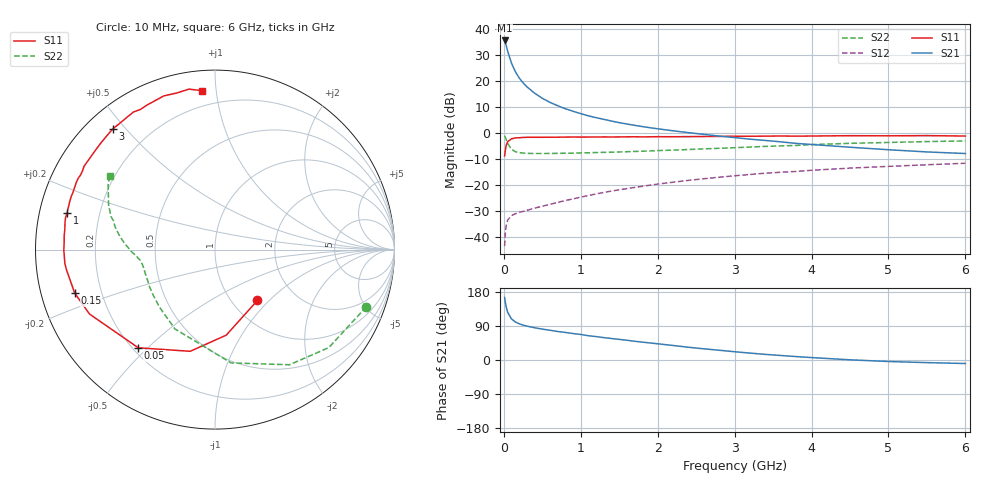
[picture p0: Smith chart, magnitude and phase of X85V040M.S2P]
! SIEMENS Small Signal Semiconductors
! BFP136W
! Si NPN RF Bipolar Junction Transistor in SOT343
! VCE = 5 V  IC = 40 mA
! Common Emitter S-Parameters:  September  1994
# GHz  S  MA  R  50
!  f  S11  S21  S12  S22
! GHz  MAG  ANG  MAG  ANG  MAG  ANG  MAG  ANG
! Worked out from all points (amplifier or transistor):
!   40 points, 10 MHz to 6 GHz, reference 50 ohm
!   highest |S21| = 35.7 dB at 10 MHz (marker M1)
!   |S21| within 3 dB of that: start of sweep to 40.07 MHz
!   unconditionally stable (mu >= 1): 746.3 MHz to 2.851 GHz
!   at 200 MHz: K = 0.48, MSG = 25.8 dB, |S12| = -30.4 dB
!   at 1.5 GHz: K = 1.11, MAG = 10.8 dB, |S12| = -21.7 dB
!   at 6 GHz: K = 0.96, MSG = 1.9 dB, |S12| = -11.5 dB
!   S11 on the Smith chart (normalised r, x): 10 MHz: 1.30, -0.85; 50 MHz: 0.22, -0.47; 150 MHz: 0.10, -0.15; 1 GHz: 0.08, +0.12; 3 GHz: 0.08, +0.46; 6 GHz: 0.11, +0.91
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0.01  0.369 -50.2  61.07 164.9  0.0068 74.4  0.9014 -20.7
0.02  0.4808 -82.5  55.19 151.4  0.0125 63.6  0.8369 -40.7
0.03  0.5832 -103.7  49.45 140.6  0.0169 55.5  0.7641 -57.1
0.05  0.6942 -128.0  37.88 125.5  0.0217 42.4  0.6377 -81.9
0.1  0.7859 -152.8  22.2 108.3  0.0263 32.7  0.4949 -116.9
0.15  0.8186 -162.8  15.33 100.3  0.0285 30.9  0.445 -134.2
0.2  0.8252 -168.3  11.6 95.5  0.0303 31.4  0.4269 -144.2
0.25  0.8353 -172.3  9.374 92.1  0.0317 32.8  0.4191 -150.7
0.3  0.84 -174.8  7.85 89.5  0.0332 34.9  0.413 -155.1
0.4  0.8422 -179.7  5.921 85.1  0.0366 38.1  0.4106 -160.9
0.5  0.8415 177.1  4.725 81.5  0.0399 41.3  0.4104 -164.6
0.6  0.8437 174.8  3.943 78.5  0.0432 43.9  0.4113 -166.9
0.8  0.849 169.9  2.973 72.7  0.0513 48.7  0.4153 -169.8
1  0.8492 166.1  2.397 67.4  0.0596 51.6  0.4209 -171.8
1.1  0.8506 163.4  2.171 64.0  0.0639 52.3  0.4244 -172.5
1.5  0.8547 156.6  1.608 54.4  0.0824 54.4  0.4394 -175.2
2.2  0.8637 144.0  1.12 38.3  0.1152 52.8  0.4765 179.8
3  0.8813 130.2  0.83 21.8  0.1534 47.6  0.5317 172.6
3.2  0.8815 126.8  0.774 18.2  0.1621 45.9  0.5459 170.5
4.5  0.9025 108.4  0.542 0.5  0.215 34.7  0.6437 157.1
5.5  0.9058 99.2  0.44 -6.9  0.2496 26.8  0.6962 148.8
6  0.8888 94.8  0.41 -9.3  0.2666 22.4  0.7151 145.2
